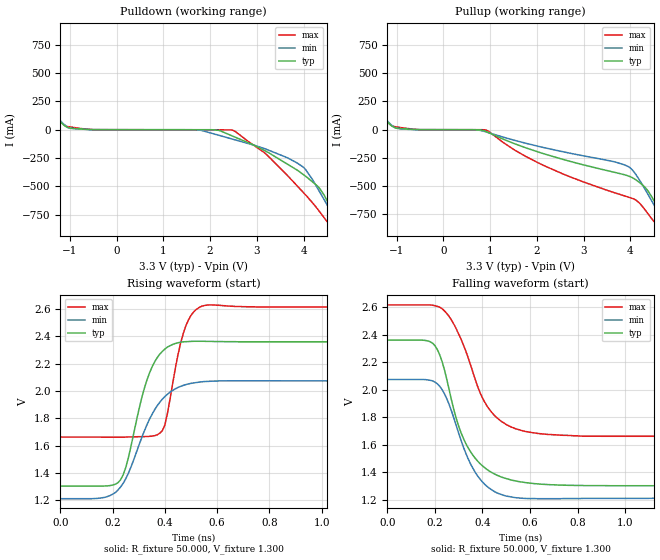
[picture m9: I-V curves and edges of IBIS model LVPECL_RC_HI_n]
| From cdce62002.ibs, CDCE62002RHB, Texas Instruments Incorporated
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|   Model LVPECL_RC_HI_n LVPECL HI SWING for UXN Pins
[Model]   LVPECL_RC_HI_n
Model_type   Output_ECL
Polarity   Non-Inverting
Enable   Active-High
Vmeas = 1.5
Vref = 0
Cref = 0
Rref = 150
|   typ   min   max
|   Strong PVT   Nominal PVT  Weak PVT
C_comp   1.8497pF   1.8465pF   1.8619pF
[Voltage Range]   3.3   3   3.6
[Temperature Range]   40   100   -40
[Pullup Reference]   3.3   3   3.6
[Pulldown Reference]   3.3   3   3.6
[Power Clamp Reference]   3.3   3   3.6
[GND Clamp Reference]   0   0   0
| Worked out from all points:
|   falling waveform, R_fixture 50.000, V_fixture 1.300: 20-80 % time 124ps typ, 118ps min, 136ps max; typ from 2.36 V to 1.3 V
|   rising waveform, R_fixture 50.000, V_fixture 1.300: 20-80 % time 84.2ps typ, 117ps min, 59.5ps max; typ from 1.3 V to 2.36 V
[Pulldown]
|   Voltage   I(typ)   I(min)   I(max)
-3.3V     1.332A     1.268A     1.428A
-2.68V    935.4mA    899.2mA    1A
-2.384V   755.4mA    723.3mA    803mA
-1.288V   115mA      119.3mA    116.2mA
-1.042V   18.84mA    20.53mA    27.56mA
1.784V    -99.23uA   -3.931mA   -1.151mA
2.483V    -56.3mA    -83.34mA   -3.998mA
3.992V    -394.4mA   -329.2mA   -551.6mA
4.342V    -515.8mA   -545.9mA   -721.8mA
4.689V    -772.5mA   -800.4mA   -915.7mA
4.89V     -944.7mA   -952.9mA   -1.1A
6.6V      -2.411A    -2.274A    -2.849A
[Pullup]
|   Voltage   I(typ)   I(min)   I(max)
-3.3V     1.332A     1.269A     1.435A
-2.63V    904.6mA    868.5mA    966.5mA
-1.489V   222.1mA    221.7mA    234.2mA
-1.067V   23.18mA    26.87mA    29.91mA
918mV     -17.38mA   -20.54mA   -4.538mA
2.059V    -201.7mA   -150mA     -300mA
3.672V    -378.5mA   -285.7mA   -559.7mA
4.02V     -420.6mA   -347.2mA   -605.4mA
4.317V    -512.5mA   -530.7mA   -711.6mA
4.689V    -772.6mA   -801mA     -911.8mA
4.838V    -894.1mA   -911.5mA   -1.037A
6.6V      -2.402A    -2.268A    -2.835A
[Ramp]
R_load = 50
|   typ   min   max
dV/dt_r   0.633591/8.41632e-11   0.517497/1.17683e-10   0.606837/5.94047e-11
dV/dt_f   0.633603/1.24459e-10   0.517459/1.1819e-10   0.6068/1.36409e-10
[Falling Waveform]
R_fixture = 50.000
V_fixture = 1.300
V_fixture_min = 1.000
V_fixture_max = 1.600
C_fixture = 0.000
|  time   V(typ)   V(min)   V(max)
0s        2.36V      2.074V     2.615V
180ps     2.348V     2.068V     2.615V
210ps     2.292V     2.043V     2.605V
240ps     2.145V     1.971V     2.572V
290ps     1.79V      1.738V     2.44V
330ps     1.609V     1.539V     2.28V
400ps     1.447V     1.33V      1.94V
480ps     1.366V     1.239V     1.769V
740ps     1.307V     1.21V      1.669V
1.7ns     1.304V     1.212V     1.663V
[Rising Waveform]
R_fixture = 50.000
V_fixture = 1.300
V_fixture_min = 1.000
V_fixture_max = 1.600
C_fixture = 0.000
|  time   V(typ)   V(min)   V(max)
0s        1.304V     1.212V     1.663V
230ps     1.35V      1.297V     1.662V
260ps     1.511V     1.398V     1.664V
330ps     2.074V     1.748V     1.667V
390ps     2.29V      1.94V      1.709V
410ps     2.322V     1.977V     1.839V
440ps     2.348V     2.016V     2.168V
490ps     2.362V     2.052V     2.52V
560ps     2.363V     2.07V      2.629V
1.7ns     2.36V      2.074V     2.615V
